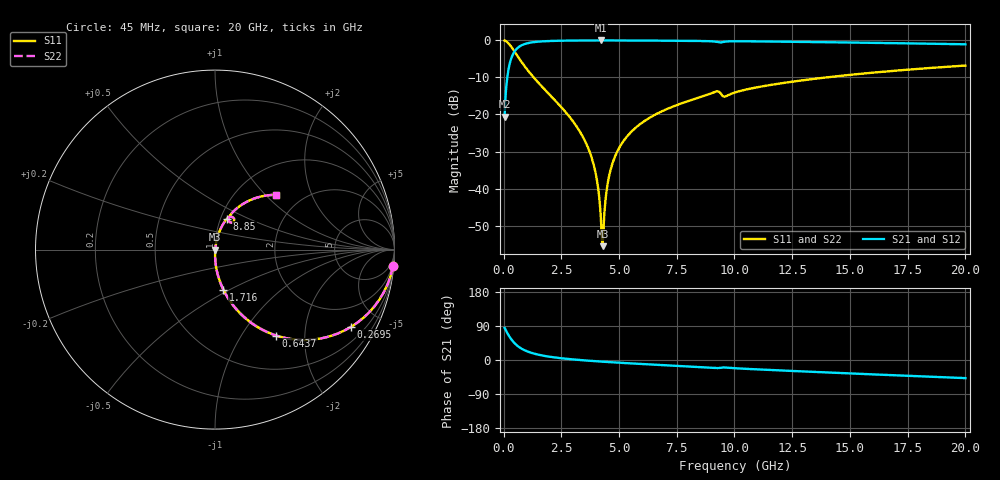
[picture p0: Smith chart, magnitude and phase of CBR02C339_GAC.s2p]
! S-parameter model data by Modelithics Inc.  support@modelithics.com 813-866-6335  Tampa FL USA
! S-Parameter data specifications:
! Substrate: 20-mil Rogers 4350B, substrate thickness, H=0.508mm, Dielectric constant, Er=3.75
! PCB Mounting Pad Footprint: Pad width, PadW=0.32mm , Pad length, PadL=0.37mm , Pad gap, PadG (edge-to-edge)=0.19mm , Reference planes=0.93mm apart
#  GHz  S  MA  R 50
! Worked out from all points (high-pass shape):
!   801 points, 45 MHz to 20 GHz, reference 50 ohm
!   highest |S21| = -0.02 dB at 4.236 GHz (marker M1); lowest = -20.6 dB at 45 MHz (marker M2)
!   |S21| within 3 dB of the highest: 474.2 MHz to end of sweep
!   lowest |S11| = -55.6 dB at 4.285 GHz (marker M3), VSWR 1.00, Z = 50.2 + j0.00354 ohm
!   |S11| at or under -10 dB: 1.305 GHz to 13.97 GHz (12.66 GHz wide, 166 % of centre)
!   |S22| runs from -55.6 to 0.0 dB; largest |S21 - S12| = 0
!   S11 on the Smith chart (normalised r, x): 45 MHz: 1, -21; 269.5 MHz: 0.98, -3.52; 643.6 MHz: 0.99, -1.45; 1.716 GHz: 0.99, -0.47; 8.85 GHz: 1.07, +0.38; 20 GHz: 1.50, +1.16
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0.045  0.9956 -5.4  0.09337 84.6  0.09337 84.6  0.9956 -5.4
0.194662  0.9263 -22.3  0.3765 67.7  0.3765 67.7  0.9263 -22.3
0.269494  0.8709 -29.7  0.491 60.3  0.491 60.3  0.8709 -29.7
0.64365  0.5886 -54.5  0.8076 35.4  0.8076 35.4  0.5886 -54.5
1.067694  0.3882 -68.1  0.9205 21.7  0.9205 21.7  0.3882 -68.1
1.716231  0.2284 -78.2  0.9723 11.4  0.9723 11.4  0.2284 -78.2
3.387462  0.05307 -88.8  0.997 -0.4  0.997 -0.4  0.05307 -88.8
3.936225  0.01903 -88.1  0.9981 -3.0  0.9981 -3.0  0.01903 -88.1
4.085888  0.01069 -84.8  0.9982 -3.6  0.9982 -3.6  0.01069 -84.8
4.23555  0.002973 -60.4  0.9983 -4.2  0.9983 -4.2  0.002973 -60.4
4.285437  0.001668 1.2  0.9983 -4.4  0.9983 -4.4  0.001668 1.2
4.360269  0.004389 62.9  0.9982 -4.7  0.9982 -4.7  0.004389 62.9
4.460044  0.009308 74.5  0.9982 -5.1  0.9982 -5.1  0.009308 74.5
4.559819  0.01425 77.7  0.9981 -5.5  0.9981 -5.5  0.01425 77.7
4.933975  0.03206 80.0  0.9977 -6.9  0.9977 -6.9  0.03206 80.0
5.6324  0.0626 79.0  0.9961 -9.4  0.9961 -9.4  0.0626 79.0
6.704981  0.1048 76.0  0.9924 -12.9  0.9924 -12.9  0.1048 76.0
8.850144  0.1857 68.6  0.9771 -19.8  0.9771 -19.8  0.1857 68.6
10.0225  0.1982 66.5  0.9739 -21.7  0.9739 -21.7  0.1982 66.5
13.36496  0.3005 58.3  0.9509 -31.2  0.9509 -31.2  0.3005 58.3
16.68248  0.3834 49.9  0.9206 -39.7  0.9206 -39.7  0.3834 49.9
20  0.4575 41.8  0.886 -47.8  0.886 -47.8  0.4575 41.8
